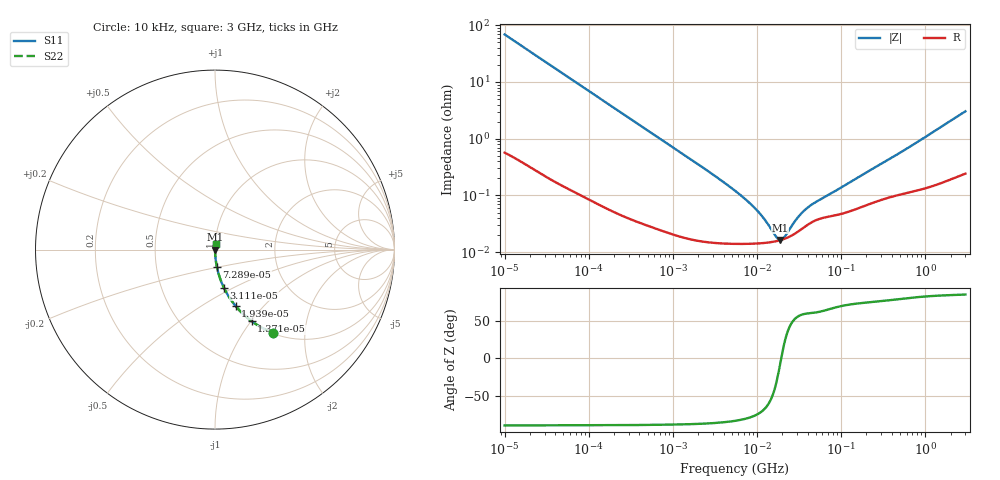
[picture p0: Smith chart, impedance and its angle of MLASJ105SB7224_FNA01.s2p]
! MLASJ105SB7224_FNA01  S-PARAMETER MODEL  ( Standard Model )
! Model Generated by TAIYO YUDEN Corporation (http://www.ty-top.com)
! Version 1.0
! TAIYO YUDEN Control No. 220601
! Copyright(c) 2009 TAIYO YUDEN CO.,LTD. All Rights Reserved.
! Product Description (link to TY-COMPAS)
! https://ds.yuden.co.jp/TYCOMPAS/or/detail?pn=MLASJ105SB7224KFNA01&u=M
! Products Name : Multilayer Ceramic Capacitors
! Characteristics :
!  Capacitance : 0.22 [uF] , Rated Voltage : 6.3 [V] , TCC : X7R
!  Case Size : 1.0 x 0.5 / 0.039 x 0.02 [mm/inch] , Thickness : 0.5 / 0.02 [mm/inch]
!  (Conditions: Temperature = 25 [degC] , DC Bias Voltage = 0 [V])
! External Node Assignments :
!  1  o---| |---o  2
! GND o---------o GND
! Frequency Range : 10kHz  -  3GHz  [ 401 STEP ]
# MHZ S RI R 50
! Freq[MHz].  S11 Real  S11 Imag  S21 Real  S21 Imag  S12 Real  S12 Imag  S22 Real  S22 Imag
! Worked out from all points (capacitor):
!   401 points, 10 kHz to 3 GHz, reference 50 ohm
!   read as one part in series: C = 231 nF near 10.65 kHz
!   lowest |Z| = 16.4 mohm at 18.73 MHz (marker M1)
!   series resonance near 19.39 MHz, so ESL is about 290 pH
!   S11 on the Smith chart (normalised r, x): 10 kHz: 1.01, -1.38; 13.71 kHz: 1.01, -1.01; 19.39 kHz: 1.01, -0.71; 31.11 kHz: 1.00, -0.45; 72.89 kHz: 1.00, -0.19; 3 GHz: 1.00, +0.06
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0.01  0.3232 -0.4636  0.6768 0.4636  0.6768 0.4636  0.3232 -0.4636
0.013707  0.2044 -0.3989  0.7956 0.3989  0.7956 0.3989  0.2044 -0.3989
0.019389  0.1152 -0.3147  0.8848 0.3147  0.8848 0.3147  0.1152 -0.3147
0.031113  0.0492 -0.2115  0.9508 0.2115  0.9508 0.2115  0.0492 -0.2115
0.072886  0.0101 -0.0946  0.9899 0.0946  0.9899 0.0946  0.0101 -0.0946
0.082683  0.00803 -0.0836  0.992 0.0836  0.992 0.0836  0.00803 -0.0836
0.199902  0.00174 -0.035  0.9983 0.035  0.9983 0.035  0.00174 -0.035
0.683653  0.000355 -0.0103  0.9996 0.0103  0.9996 0.0103  0.000355 -0.0103
2.570001  0.000157 -0.00273  0.9998 0.00273  0.9998 0.00273  0.000157 -0.00273
5.477226  0.000141 -0.0012  0.9999 0.0012  0.9999 0.0012  0.000141 -0.0012
7.747855  0.000141 -0.000778  0.9999 0.000778  0.9999 0.000778  0.000141 -0.000778
9.97066  0.000142 -0.00053  0.9999 0.00053  0.9999 0.00053  0.000142 -0.00053
12.43293  0.000146 -0.000341  0.9999 0.000341  0.9999 0.000341  0.000146 -0.000341
17.04125  0.000156 -9.63e-05  0.9998 9.63e-05  0.9998 9.63e-05  0.000156 -9.63e-05
18.73182  0.000162 -2.58e-05  0.9998 2.58e-05  0.9998 2.58e-05  0.000162 -2.58e-05
19.95104  0.000166 2.1e-05  0.9998 -2.1e-05  0.9998 -2.1e-05  0.000166 2.1e-05
21.24962  0.000172 6.78e-05  0.9998 -6.78e-05  0.9998 -6.78e-05  0.000172 6.78e-05
28.22191  0.000212 0.00028  0.9998 -0.00028  0.9998 -0.00028  0.000212 0.00028
33.04079  0.000248 0.000396  0.9998 -0.000396  0.9998 -0.000396  0.000248 0.000396
45.28751  0.00034 0.000609  0.9997 -0.000609  0.9997 -0.000609  0.00034 0.000609
374.4521  0.000939 0.00427  0.9991 -0.00427  0.9991 -0.00427  0.000939 0.00427
3000  0.00333 0.0302  0.9967 -0.0302  0.9967 -0.0302  0.00333 0.0302
